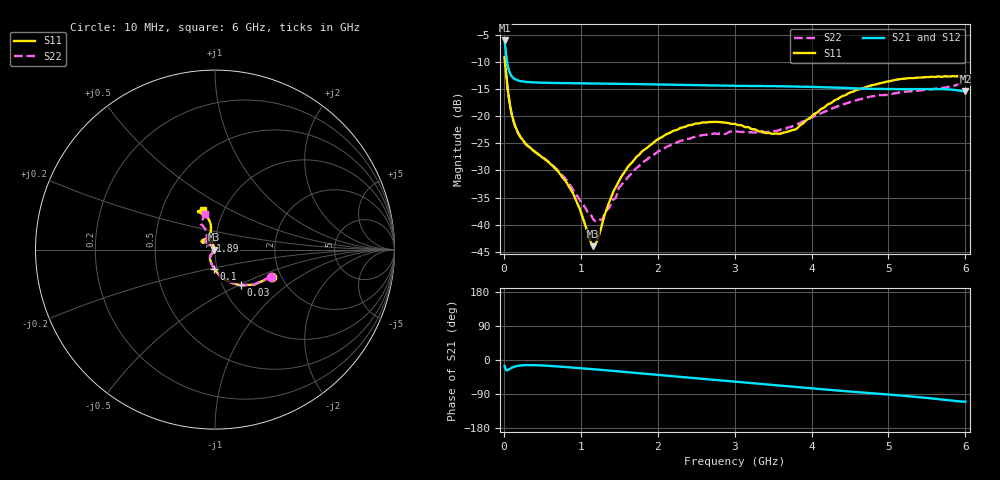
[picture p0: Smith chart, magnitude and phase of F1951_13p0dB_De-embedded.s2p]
! Integrated Device Technology
! Corporate Headquarters
! 6024 Silver Creek Valley Road
! San Jose, CA 95138  USA
! Phone:  1-408-284-8200
! Toll Free:  1-800-223-1366
! Webpage:  http://www.idt.com/
! Timing and RF Division
! 515 Groton Road, Suite 102
! Westford, MA 01886-6024
! Device:  F1951
! Description: 6-bit 0.5 dB Digital Step Attenuator
! Frequency:  100.0 -  4000.00 MHz
! Package:  4x4 mm Thin QFN Plastic Package: 24 pin
! Ports:  2 RF, 6 DC
!  Pin  1  = NC
!  Pin  2  = RF1  =  Port 1
!  Pin  3  = GND
!  Pin  4  = NC
!  Pin  5  = Serial Data Out (SDO)
!  Pin  6  = NC
!  Pin  7  = Reset Bar ( RSTb)
!  Pin  8  = Clock (CLK)
!  Pin  9  = Chip Select Bar (CSb)
!  Pin 10  = NC
!  Pin 11  = Serial Data In (SDI)
!  Pin 12  = NC
!  Pin 13  = NC
!  Pin 14  = VDD
!  Pin 15  = NC
!  Pin 16  = GND
!  Pin 17  = RF2  =  Port 2
!  Pin 18  = NC
!  Pin 19  = GND
!  Pin 20  = GND
!  Pin 21  = GND
!  Pin 22  = GND
!  Pin 23  = GND
!  Pin 24  = GND
! State:  26
! Atten State:  13.0 dB
! Voltage:  +3.30 Volts
! Current:  0.476 mA
! Data:  The device was measured on a F195X evaluation board which has
!  individual transmission lines to the RF pins.  Data was collected
!  de-embedded using a Automatic Fixture Removal [AFR] (Keysight Technologies).
!  The reference plane is the edge of the package pin.
! Misc:  Lot Code  1225BCA
!  Action Tracker AT0399
! Date Measured:  2018-09-13
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# GHz S dB R 50
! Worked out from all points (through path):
!   600 points, 10 MHz to 6 GHz, reference 50 ohm
!   highest |S21| = -6.02 dB at 10 MHz (marker M1); lowest = -15.4 dB at 6 GHz (marker M2)
!   group delay of S21, straight-line fit = 47 ps
!   lowest |S11| = -44.0 dB at 1.16 GHz (marker M3), VSWR 1.01, Z = 49.4 + j0.00339 ohm
!   |S11| at or under -10 dB: 15.74 MHz to end of sweep
!   |S22| runs from -39.4 to -9.2 dB; largest |S21 - S12| = 0.00038
!   S11 on the Smith chart (normalised r, x): 10 MHz: 1.79, -0.62; 30 MHz: 1.22, -0.52; 100 MHz: 0.97, -0.21; 1.89 GHz: 0.94, +0.09; 6 GHz: 0.80, +0.37
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0.01  -9.11 -25.7  -6.02 -15.7  -6.02 -15.7  -9.18 -25.9
0.03  -12.19 -54.1  -8.66 -26.5  -8.66 -26.5  -12.28 -54.4
0.06  -16.05 -76.4  -11.21 -25.8  -11.22 -25.8  -16.16 -76.9
0.1  -19.42 -92.3  -12.58 -20.8  -12.58 -20.8  -19.50 -92.9
0.17  -22.59 -107.8  -13.33 -15.9  -13.33 -15.9  -22.72 -108.4
0.26  -24.65 -117.8  -13.62 -13.7  -13.62 -13.7  -24.81 -118.9
0.72  -30.45 -123.8  -13.88 -17.2  -13.88 -17.2  -30.25 -129.4
0.88  -33.74 -124.7  -13.92 -19.7  -13.92 -19.7  -33.09 -131.5
1.01  -38.04 -130.8  -13.95 -21.8  -13.95 -21.8  -35.98 -137.0
1.16  -43.97 179.7  -13.97 -24.2  -13.97 -24.2  -38.92 -161.0
1.21  -43.04 151.2  -13.97 -25.0  -13.98 -25.1  -39.13 -175.6
1.28  -39.79 125.7  -13.98 -26.3  -13.98 -26.3  -38.98 165.6
1.51  -31.59 111.9  -14.03 -30.2  -14.03 -30.2  -32.96 135.7
1.89  -25.50 119.9  -14.11 -37.2  -14.11 -37.2  -27.57 132.6
2.01  -24.18 124.0  -14.14 -39.4  -14.14 -39.4  -26.44 135.1
2.49  -21.36 139.0  -14.26 -48.0  -14.26 -48.0  -23.78 144.9
3.01  -21.43 150.3  -14.38 -57.2  -14.39 -57.2  -22.79 149.3
3.58  -23.25 129.5  -14.46 -67.3  -14.46 -67.3  -22.54 131.2
4.01  -19.89 103.5  -14.58 -75.0  -14.58 -75.0  -20.19 117.8
4.49  -15.69 100.8  -14.81 -83.2  -14.81 -83.2  -17.43 116.1
5.01  -13.56 109.6  -15.00 -91.2  -15.00 -91.2  -16.03 118.7
6  -12.79 106.6  -15.42 -110.1  -15.42 -110.0  -13.79 106.1
